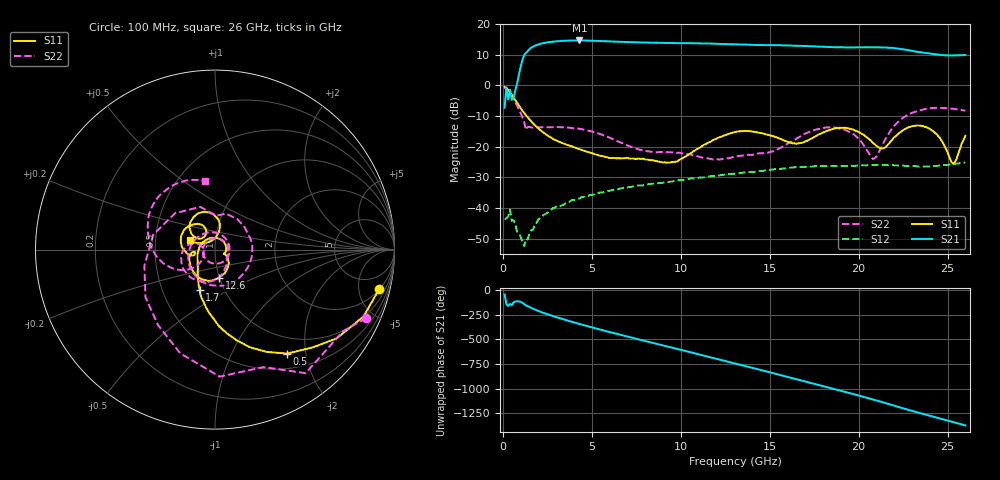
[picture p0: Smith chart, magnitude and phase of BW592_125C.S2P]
!Keysight Technologies,N5247A,US51370447,A.10.64.09
!Date: Thursday, March 05, 2020 07:26:41
!Correction: S11(Full 2 Port with power(1,2))
!S21(Full 2 Port with power(1,2))
!S12(Full 2 Port with power(1,2))
!S22(Full 2 Port with power(1,2))
!S2P File: Measurements: S11, S21, S12, S22:
# Hz S  dB  R 50
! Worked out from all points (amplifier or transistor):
!   260 points, 100 MHz to 26 GHz, reference 50 ohm
!   highest |S21| = 14.7 dB at 4.3 GHz (marker M1)
!   |S21| within 3 dB of that: 1.471 GHz to 22.61 GHz (21.14 GHz wide, 176 % of centre)
!   unconditionally stable (mu >= 1): start of sweep to end of sweep
!   at 4.4 GHz: K = 5.97, MAG = 14.9 dB, |S12| = -36.6 dB
!   at 13.1 GHz: K = 2.88, MAG = 13.6 dB, |S12| = -28.7 dB
!   at 26 GHz: K = 2.47, MAG = 10.8 dB, |S12| = -25.1 dB
!   S11 on the Smith chart (normalised r, x): 100 MHz: 2.08, -7.99; 500 MHz: 0.73, -1.67; 1.7 GHz: 0.77, -0.37; 12.6 GHz: 0.99, -0.32; 26 GHz: 0.75, +0.08
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1e8  -0.52 -13.4  -7.26 -46.6  -43.71 0.6  -0.68 -24.4
5e8  -3.03 -55.2  -4.65 -154.2  -44.24 -24.8  -3.00 -87.8
1.1e9  -8.25 -91.0  8.34 -130.6  -51.18 -42.9  -10.44 137.5
1.7e9  -12.39 -110.7  12.68 168.5  -47.10 16.9  -13.82 25.7
2.9e9  -17.70 -137.0  14.36 89.9  -39.97 -14.4  -13.66 -46.9
4.3e9  -20.76 179.9  14.70 15.1  -36.96 -57.2  -14.16 -104.2
4.5e9  -21.17 170.9  14.69 5.1  -36.39 -63.9  -14.34 -112.7
5.5e9  -23.01 122.2  14.52 -43.7  -34.88 -98.2  -15.94 -158.4
6.5e9  -23.80 65.9  14.28 -90.0  -33.84 -131.7  -18.33 148.9
7.8e9  -23.97 7.9  14.04 -148.8  -32.73 -178.0  -21.10 63.3
8.8e9  -24.93 -20.2  13.94 166.3  -31.84 143.9  -21.71 -10.9
1.06e10  -22.01 -31.0  13.79 85.3  -30.29 71.6  -22.64 -135.0
1.26e10  -15.99 -82.0  13.52 -5.8  -29.08 -11.8  -23.77 73.1
1.31e10  -15.18 -98.0  13.44 -28.6  -28.73 -33.0  -23.19 39.7
1.49e10  -16.09 -154.2  13.18 -110.2  -27.61 -107.4  -21.94 -33.1
1.61e10  -18.53 -173.5  13.07 -166.4  -26.90 -156.3  -18.77 -60.0
1.74e10  -17.18 -167.1  12.81 132.6  -26.51 148.4  -14.73 -101.5
1.86e10  -14.13 166.0  12.51 75.8  -26.34 96.9  -13.71 -148.7
1.99e10  -14.94 127.5  12.44 14.2  -26.19 39.9  -16.85 167.5
2.17e10  -19.00 146.7  12.30 -78.1  -26.01 -48.4  -15.62 -140.9
2.36e10  -13.26 104.7  10.76 -176.9  -26.48 -144.9  -7.90 158.0
2.6e10  -16.41 159.4  9.95 65.5  -25.11 101.4  -8.27 98.6
